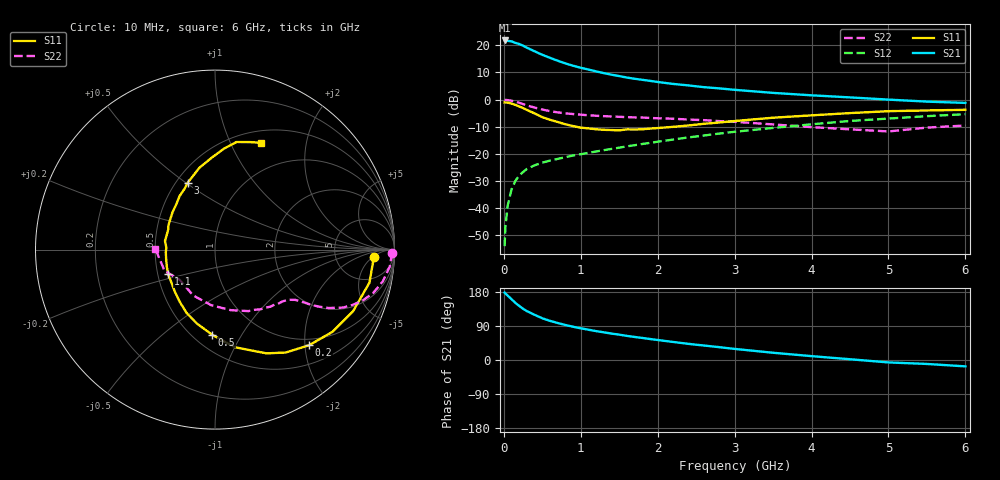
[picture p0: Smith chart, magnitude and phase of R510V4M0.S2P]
! SIEMENS Small Signal Semiconductors
! BFR183
! Si NPN RF Bipolar Junction Transistor in SOT23
! VCE = 10 V  IC = 4 mA
! Common Emitter S-Parameters:  May  1996
# GHz  S  MA  R  50
!  f  S11  S21  S12  S22
! GHz  MAG  ANG  MAG  ANG  MAG  ANG  MAG  ANG
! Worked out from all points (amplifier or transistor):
!   36 points, 10 MHz to 6 GHz, reference 50 ohm
!   highest |S21| = 21.8 dB at 10 MHz (marker M1)
!   |S21| within 3 dB of that: start of sweep to 324.9 MHz
!   unconditionally stable (mu >= 1): 1.197 GHz to 2.789 GHz
!   at 250 MHz: K = 0.35, MSG = 23.3 dB, |S12| = -26.7 dB
!   at 1.4 GHz: K = 1.05, MAG = 12.4 dB, |S12| = -18.2 dB
!   at 6 GHz: K = 0.87, MSG = 2.1 dB, |S12| = -5.4 dB
!   S11 on the Smith chart (normalised r, x): 10 MHz: 15, -5; 200 MHz: 0.86, -2.09; 500 MHz: 0.62, -0.75; 1.1 GHz: 0.57, -0.17; 3 GHz: 0.57, +0.51; 6 GHz: 0.64, +1.31
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0.01  0.8851 -2.5  12.26 177.9  0.002 86.7  0.9884 -1.0
0.02  0.8829 -4.8  12.08 175.6  0.0045 82.1  0.9839 -2.3
0.05  0.88 -12.1  12.04 169.9  0.0112 83.6  0.9785 -5.5
0.1  0.8424 -24.0  11.82 160.4  0.0222 76.5  0.9517 -10.7
0.15  0.7984 -35.1  11.07 150.8  0.0318 71.2  0.9141 -15.3
0.2  0.7472 -45.5  10.53 142.7  0.04 66.9  0.8719 -18.9
0.25  0.6958 -55.5  9.813 135.2  0.0464 63.3  0.8249 -22.0
0.3  0.6454 -63.6  9.015 129.0  0.0529 60.3  0.7821 -24.4
0.4  0.5551 -78.5  7.735 119.2  0.0616 56.5  0.7123 -27.2
0.5  0.4742 -92.0  6.672 110.1  0.069 54.3  0.6556 -28.9
0.6  0.4243 -103.7  5.87 103.3  0.0753 53.7  0.6123 -30.0
0.7  0.3865 -114.2  5.192 97.6  0.0809 53.4  0.5812 -30.6
0.8  0.3508 -124.1  4.631 92.4  0.0869 53.3  0.5577 -31.2
1.1  0.2947 -152.7  3.568 79.9  0.1045 54.7  0.5141 -33.0
1.3  0.2776 -168.5  3.068 73.0  0.1173 55.7  0.4948 -34.4
1.6  0.2827 170.3  2.543 63.6  0.1376 56.3  0.4739 -37.5
2.2  0.3148 138.8  1.941 47.6  0.1835 55.8  0.444 -45.7
3  0.4028 112.1  1.512 29.3  0.2552 51.3  0.3899 -61.5
3.5  0.4635 100.9  1.328 19.1  0.3005 46.5  0.3487 -75.4
4.5  0.564 85.0  1.097 2.0  0.404 35.6  0.283 -115.5
5.5  0.6308 71.7  0.917 -10.4  0.4951 23.4  0.305 -157.2
6  0.648 66.6  0.868 -16.8  0.5383 15.3  0.333 179.0
